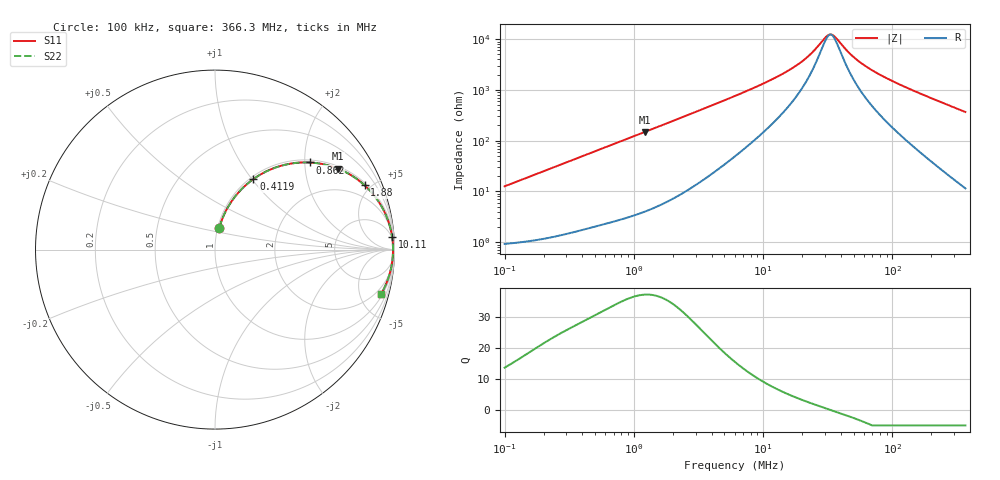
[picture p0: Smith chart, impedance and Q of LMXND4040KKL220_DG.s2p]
! LMXND4040KKL220_DG  S-PARAMETER MODEL  ( General Type )
! Model Generated by TAIYO YUDEN Corporation (https://www.yuden.co.jp/en/)
! Version 1.0
! TAIYO YUDEN Control No. 191023NI43SB-FBB
! Copyright(c) 2019 TAIYO YUDEN CO.,LTD. All Rights Reserved.
! Product Description (link to TY-COMPAS)
! https://ds.yuden.co.jp/TYCOMPAS/or/detail?pn=LMXND4040KKL220MDG&u=M
! Products Name : Inductors
! Characteristics :
!  Inductance : 22 uH , SRF(min) : 19 MHz , DC Resistance(max) : 0.684 Ohm
!  Rated Current : Saturation :450 mA , Temp Rise : 500 mA (40 degC)
!  Case Size : 4.0 x 4.0 / 0.157 x 0.157 [mm/inch] , Thickness : 1 / 0.039 [mm/inch]
!  (Conditions: Temperature = 25 degC , DC Bias Current/Voltage = 0A / 0V)
! External Node Assignments :
!  1  o---GGG---o  2
! GND o---------o GND
! Frequency Range : 0.1MHz  -  366.261039MHz  [ 402 STEP ]
# MHz S RI R 50
! Freq[MHz].  S11 Real  S11 Imag  S21 Real  S21 Imag  S12 Real  S12 Imag  S22 Real  S22 Imag
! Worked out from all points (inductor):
!   401 points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, 100 kHz to 366.3 MHz, reference 50 ohm
!   read as one part in series: L = 20 uH near 104.2 kHz
!   highest Q = 37.1 at 1.222 MHz (marker M1), where L = 19.5 uH
!   self-resonance near 32.54 MHz
!   S11 on the Smith chart (normalised r, x): 100 kHz: 1.02, +0.25; 411.9 kHz: 1.04, +1.02; 862 kHz: 1.06, +2.11; 1.88 MHz: 1.13, +4.60; 10.11 MHz: 4, +27; 366.3 MHz: 1.23, -7.36
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0.1  0.0243 0.1217  0.9757 -0.1217  0.9757 -0.1217  0.0243 0.1217
0.218052  0.0785 0.2476  0.9215 -0.2476  0.9215 -0.2476  0.0785 0.2476
0.395307  0.2017 0.3839  0.7983 -0.3839  0.7983 -0.3839  0.2017 0.3839
0.411864  0.2143 0.3932  0.7857 -0.3932  0.7857 -0.3932  0.2143 0.3932
0.620788  0.3723 0.4683  0.6277 -0.4683  0.6277 -0.4683  0.3723 0.4683
0.861976  0.5269 0.4854  0.4731 -0.4854  0.4731 -0.4854  0.5269 0.4854
1.221676  0.6862 0.4508  0.3138 -0.4508  0.3138 -0.4508  0.6862 0.4508
1.562679  0.7788 0.4016  0.2212 -0.4016  0.2212 -0.4016  0.7788 0.4016
1.879556  0.8339 0.3581  0.1661 -0.3581  0.1661 -0.3581  0.8339 0.3581
3.139006  0.9292 0.2384  0.0708 -0.2384  0.0708 -0.2384  0.9292 0.2384
6.177387  0.9758 0.1241  0.0242 -0.1241  0.0242 -0.1241  0.9758 0.1241
10.10723  0.9866 0.0721  0.0134 -0.0721  0.0134 -0.0721  0.9866 0.0721
16.87987  0.9907 0.0354  0.00931 -0.0354  0.00931 -0.0354  0.9907 0.0354
23.92381  0.9917 0.0162  0.00829 -0.0162  0.00829 -0.0162  0.9917 0.0162
30.60159  0.992 0.00389  0.00803 -0.00389  0.00803 -0.00389  0.992 0.00389
33.90716  0.992 -0.00112  0.00801 0.00112  0.00801 0.00112  0.992 -0.00112
36.05951  0.992 -0.00412  0.00803 0.00412  0.00803 0.00412  0.992 -0.00412
45.1881  0.9918 -0.0154  0.00824 0.0154  0.00824 0.0154  0.9918 -0.0154
54.35123  0.9914 -0.0251  0.00864 0.0251  0.00864 0.0251  0.9914 -0.0251
94.57258  0.9882 -0.0608  0.0118 0.0608  0.0118 0.0608  0.9882 -0.0608
189.9711  0.9737 -0.133  0.0263 0.133  0.0263 0.133  0.9737 -0.133
366.261  0.9245 -0.249  0.0755 0.249  0.0755 0.249  0.9245 -0.249
